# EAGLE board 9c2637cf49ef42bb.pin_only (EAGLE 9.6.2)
REV: D

Size 62.48 x 81.28 mm. Coordinates in mm from the lower left corner, seen from the top.
Outline: 0,2.54 arc90 2.54,0 59.94,0 arc90 62.48,2.54 arc90 59.94,5.08 56.64,5.08 56.64,76.2 59.94,76.2 arc90 62.48,78.74 arc90 59.94,81.28 2.54,81.28 arc90 0,78.74 arc90 2.54,76.2 5.84,76.2 5.84,5.08 2.54,5.08 arc90 0,2.54
Outline: 16.26,24.89 16.26,19.56 37.21,19.56 37.21,6.1 53.21,6.1 53.21,19.56 46.23,19.56 46.23,24.89 16.26,24.89
Copper layers (1*16): Top 0.035mm / dielectric 1.5mm / Bottom 0.035mm
Design rules "adafruit *": minimum track width 8mil, minimum drill 15.5mil, track to track 8mil, track to pad 8mil, pad to pad 8mil, via to via 8mil, smd to smd 8mil, copper to edge 10mil, drill to drill 8mil, minimum pad ring 10mil, minimum via ring 8mil, stop-mask expansion 4mil, vias tented up to drill 20mil, thermal gap 10mil
tRestrict: area 42.7,32.6 to 42.8,32.9; area 43.2,32.6 to 43.3,32.9

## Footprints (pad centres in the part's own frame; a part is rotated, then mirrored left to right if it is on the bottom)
0805-NO = smd 1.24 x 1.5: 1 -0.95,0; 2 0.95,0
TFT_2.83IN_240X320_50PIN = smd 0.275 x 1.2 bottom: 1 12.25,1.04; 2 11.75,1.04; 3 11.25,1.04; 4 10.75,1.04; 5 10.25,1.04; 6 9.75,1.04; 7 9.25,1.04; 8 8.75,1.04; 9 8.25,1.04; 10 7.75,1.04; 11 7.25,1.04; 12 6.75,1.04; 13 6.25,1.04; 14 5.75,1.04; 15 5.25,1.04; 16 4.75,1.04; 17 4.25,1.04; 18 3.75,1.04; 19 3.25,1.04; 20 2.75,1.04; 21 2.25,1.04; 22 1.75,1.04; 23 1.25,1.04; 24 0.75,1.04; 25 0.25,1.04; 26 -0.25,1.04; 27 -0.75,1.04; 28 -1.25,1.04; 29 -1.75,1.04; 30 -2.25,1.04; 31 -2.75,1.04; 32 -3.25,1.04; 33 -3.75,1.04; 34 -4.25,1.04; 35 -4.75,1.04; 36 -5.25,1.04; 37 -5.75,1.04; 38 -6.25,1.04; 39 -6.75,1.04; 40 -7.25,1.04; 41 -7.75,1.04; 42 -8.25,1.04; 43 -8.75,1.04; 44 -9.25,1.04; 45 -9.75,1.04; 46 -10.25,1.04; 47 -10.75,1.04; 48 -11.25,1.04; 49 -11.75,1.04; 50 -12.25,1.04 | smd 2.54 x 3.81 bottom: PAD1 14.35,-1.152; PAD2 -14.35,-1.152
SOT23-WIDE = smd 1 x 1.2: 1 -0.95,-1; 2 0.95,-1; 3 0,1
1X20_ROUND = drill 1 pad 1.676: 1 -24.13,0; 2 -21.59,0; 3 -19.05,0; 4 -16.51,0; 5 -13.97,0; 6 -11.43,0; 7 -8.89,0; 8 -6.35,0; 9 -3.81,0; 10 -1.27,0; 11 1.27,0; 12 3.81,0; 13 6.35,0; 14 8.89,0; 15 11.43,0; 16 13.97,0; 17 16.51,0; 18 19.05,0; 19 21.59,0; 20 24.13,0
0603-NO = smd 1.075 x 1: 1 -0.85,0; 2 0.85,0
SOLDERJUMPER_ARROW_NOPASTE = smd 0.762 x 1.524: 1 -1.016,0; 2 1.016,0
TP06R = smd 0.6 x 0.6: TP 0,0
SOT23-5 = smd 0.55 x 1.2: 1 -0.95,-1.3; 2 0,-1.3; 3 0.95,-1.3; 4 0.95,1.3; 5 -0.95,1.3
TSSOP20 = smd 0.305 x 0.991: 1 -2.925,-2.918; 2 -2.275,-2.918; 3 -1.625,-2.918; 4 -0.975,-2.918; 5 -0.325,-2.918; 6 0.325,-2.918; 7 0.975,-2.918; 8 1.625,-2.918; 9 2.275,-2.918; 10 2.925,-2.918; 11 2.925,2.918; 12 2.275,2.918; 13 1.625,2.918; 14 0.975,2.918; 15 0.325,2.918; 16 -0.325,2.918; 17 -0.975,2.918; 18 -1.625,2.918; 19 -2.275,2.918; 20 -2.925,2.918
MOUNTINGHOLE_3.0_PLATEDTHIN = drill 3 pad 3.6: P$1 0,0
FIDUCIAL_1MM = smd 1 x 1: 1 0,0
EYE_SPI_DISPLAY_BOTCONTACT = smd 0.25 x 1.4: 1 4.25,1.154; 2 3.75,1.154; 3 3.25,1.154; 4 2.75,1.154; 5 2.25,1.154; 6 1.75,1.154; 7 1.25,1.154; 8 0.75,1.154; 9 0.25,1.154; 10 -0.25,1.154; 11 -0.75,1.154; 12 -1.25,1.154; 13 -1.75,1.154; 14 -2.25,1.154; 15 -2.75,1.154; 16 -3.25,1.154; 17 -3.75,1.154; 18 -4.25,1.154 | smd 1.8 x 3.5: SUPPORT1 -5.8,-1.152; SUPPORT2 5.8,-1.152
MICROSD = smd 0.7 x 1.5: 1 1.761,-3.147; 2 0.661,-2.747; 3 -0.439,-3.147; 4 -1.539,-3.547; 5 -2.639,-3.147; 6 -3.739,-3.547; 7 -4.839,-3.147; 8 -5.939,-3.147 | smd 1.8 x 1.4: CD1 -5.239,7.053; CD2 0.38,7.053 | smd 1.4 x 1.9: MT1 -6.839,-6.047; MT2 6.361,-6.947

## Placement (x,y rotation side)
C1  10uF  [0805-NO]  16.26,50.8 0 top
C3  10uF  [0805-NO]  50.04,44.32 0 top
C4  10uF  [0805-NO]  25.91,38.35 270 top
C5  10uF  [0805-NO]  51.44,37.08 270 top
CONN1  2.8" CTP ILI9341  [TFT_2.83IN_240X320_50PIN]  31.24,31.75 0 bottom
IC4  APX803-SAG  [SOT23-WIDE]  36.32,49.78 0 top
JP1  [1X20_ROUND]  31.24,78.74 180 top
JP2  [1X20_ROUND]  31.24,2.54 180 top
PLABEL0  [PLABEL0]  27.43,37.97 0 top
PLABEL1  [PLABEL1]  55.88,17.65 90 top
PLABEL2  [PLABEL2]  26.54,52.7 0 top
PLABEL3  [PLABEL3]  24.64,65.28 0 top
PLABEL4  [PLABEL4]  6.6,77.47 270 top
PLABEL5  [PLABEL5]  8.89,77.47 270 top
PLABEL6  [PLABEL6]  11.43,77.47 270 top
PLABEL7  [PLABEL7]  13.97,77.6 270 top
PLABEL8  [PLABEL8]  16.64,77.72 270 top
PLABEL9  [PLABEL9]  19.18,77.72 270 top
PLABEL10  [PLABEL10]  21.59,77.72 270 top
PLABEL11  [PLABEL11]  24.26,77.72 270 top
PLABEL12  [PLABEL12]  26.8,77.72 270 top
PLABEL13  [PLABEL13]  29.21,77.72 270 top
PLABEL14  [PLABEL14]  31.88,77.72 270 top
PLABEL15  [PLABEL15]  34.29,77.72 270 top
PLABEL16  [PLABEL16]  36.96,77.72 270 top
PLABEL17  [PLABEL17]  39.5,77.72 270 top
PLABEL18  [PLABEL18]  41.91,77.72 270 top
PLABEL19  [PLABEL19]  44.58,77.72 270 top
PLABEL20  [PLABEL20]  47.12,77.72 270 top
PLABEL21  [PLABEL21]  49.53,77.6 270 top
PLABEL22  [PLABEL22]  52.2,77.72 270 top
PLABEL23  [PLABEL23]  54.61,77.72 270 top
PLABEL24  [PLABEL24]  11.18,67.56 0 top
PLABEL25  [PLABEL25]  27.81,68.33 0 top
PLABEL26  [PLABEL26]  39.62,69.85 0 top
PLABEL27  [PLABEL27]  52.58,69.6 0 top
PLABEL28  [PLABEL28]  39.62,68.2 0 top
PLABEL29  [PLABEL29]  11.43,69.6 0 top
PLABEL30  [PLABEL30]  27.3,34.67 0 top
PLABEL31  [PLABEL31]  7.62,3.81 90 top
PLABEL32  [PLABEL32]  10.16,3.81 90 top
PLABEL33  [PLABEL33]  12.7,3.81 90 top
PLABEL34  [PLABEL34]  15.24,3.81 90 top
PLABEL35  [PLABEL35]  17.78,3.81 90 top
PLABEL36  [PLABEL36]  20.32,3.81 90 top
PLABEL37  [PLABEL37]  22.86,3.81 90 top
PLABEL38  [PLABEL38]  25.4,3.81 90 top
PLABEL39  [PLABEL39]  27.94,3.81 90 top
PLABEL40  [PLABEL40]  30.48,3.81 90 top
PLABEL41  [PLABEL41]  33.02,3.81 90 top
PLABEL42  [PLABEL42]  35.56,3.81 90 top
PLABEL43  [PLABEL43]  38.1,3.68 90 top
PLABEL44  [PLABEL44]  40.51,3.68 90 top
PLABEL45  [PLABEL45]  40.89,3.68 0 top
PLABEL46  [PLABEL46]  43.43,0.38 0 top
PLABEL47  [PLABEL47]  46.23,3.68 0 top
PLABEL48  [PLABEL48]  50.8,3.43 90 top
PLABEL49  [PLABEL49]  53.34,3.56 90 top
PLABEL50  [PLABEL50]  56.01,3.56 90 top
PLABEL51  [PLABEL51]  7.75,30.99 0 top
PLABEL52  [PLABEL52]  7.87,34.8 0 top
PLABEL53  [PLABEL53]  7.75,38.73 0 top
PLABEL54  [PLABEL54]  7.75,42.8 0 top
PLABEL55  [PLABEL55]  28.58,14.86 0 top
PLABEL56  [PLABEL56]  13.84,28.96 90 top
PLABEL57  [PLABEL57]  9.65,77.47 0 bottom
PLABEL58  [PLABEL58]  12.19,77.47 0 bottom
PLABEL59  [PLABEL59]  14.73,77.47 0 bottom
PLABEL60  [PLABEL60]  17.27,77.47 0 bottom
PLABEL61  [PLABEL61]  7.11,77.47 0 bottom
PLABEL62  [PLABEL62]  19.81,77.47 0 bottom
PLABEL63  [PLABEL63]  22.35,77.47 0 bottom
PLABEL64  [PLABEL64]  24.89,77.47 0 bottom
PLABEL65  [PLABEL65]  27.3,81.03 0 bottom
PLABEL66  [PLABEL66]  29.97,77.47 0 bottom
PLABEL67  [PLABEL67]  32.64,81.03 0 bottom
PLABEL68  [PLABEL68]  35.05,77.47 0 bottom
PLABEL69  [PLABEL69]  37.59,81.15 0 bottom
PLABEL70  [PLABEL70]  40.13,77.47 0 bottom
PLABEL71  [PLABEL71]  42.8,79.88 180 bottom
PLABEL72  [PLABEL72]  45.21,77.47 0 bottom
PLABEL73  [PLABEL73]  47.62,79.76 180 bottom
PLABEL74  [PLABEL74]  50.29,77.47 0 bottom
PLABEL75  [PLABEL75]  52.83,81.15 0 bottom
PLABEL76  [PLABEL76]  55.37,77.6 0 bottom
PLABEL77  [PLABEL77]  7.11,5.08 0 bottom
PLABEL78  [PLABEL78]  9.65,0.25 0 bottom
PLABEL79  [PLABEL79]  12.19,3.68 0 bottom
PLABEL80  [PLABEL80]  14.73,0.25 0 bottom
PLABEL81  [PLABEL81]  17.27,3.68 0 bottom
PLABEL82  [PLABEL82]  19.81,0.25 0 bottom
PLABEL83  [PLABEL83]  22.35,3.68 0 bottom
PLABEL84  [PLABEL84]  24.89,0.25 0 bottom
PLABEL85  [PLABEL85]  27.43,3.68 0 bottom
PLABEL86  [PLABEL86]  29.97,0.25 0 bottom
PLABEL87  [PLABEL87]  32.51,3.68 0 bottom
PLABEL88  [PLABEL88]  35.05,0.25 0 bottom
PLABEL89  [PLABEL89]  37.59,3.56 0 bottom
PLABEL90  [PLABEL90]  40.26,0.25 0 bottom
PLABEL91  [PLABEL91]  42.67,3.68 0 bottom
PLABEL92  [PLABEL92]  45.09,0.25 0 bottom
PLABEL93  [PLABEL93]  47.75,3.68 0 bottom
PLABEL94  [PLABEL94]  50.29,0.25 0 bottom
PLABEL95  [PLABEL95]  52.83,3.56 0 bottom
PLABEL96  [PLABEL96]  55.37,0.25 0 bottom
Q2  BSS138  [SOT23-WIDE]  22.35,10.92 180 top
Q3  BSS138  [SOT23-WIDE]  26.29,10.92 180 top
Q4  BSS138  [SOT23-WIDE]  14.48,37.47 0 top
R1  10  [0603-NO]  17.53,38.35 270 top
R2  10  [0603-NO]  19.56,38.35 270 top
R3  10  [0603-NO]  21.59,38.35 270 top
R4  10  [0603-NO]  23.62,38.35 270 top
R5  2.2K  [0603-NO]  14.22,40.89 180 top
R6  10K  [0603-NO]  38.86,49.78 90 top
R7  1K  [0603-NO]  37.85,68.07 0 top
R8  10K  [0603-NO]  8.76,13.21 90 top
R9  10K  [0603-NO]  11.18,12.57 90 top
R10  10K  [0603-NO]  16.38,12.57 270 top
R11  10K  [0603-NO]  13.72,12.57 270 top
R12  10K  [0603-NO]  37.47,62.87 270 top
R13  10K  [0603-NO]  22.48,8.26 0 top
R14  10K  [0603-NO]  26.29,8.26 180 top
R15  10K  [0603-NO]  26.29,13.72 180 top
R16  10K  [0603-NO]  22.35,13.72 0 top
SJ1  [SOLDERJUMPER_ARROW_NOPASTE]  8.89,29.72 180 top
SJ2  [SOLDERJUMPER_ARROW_NOPASTE]  8.89,33.53 180 top
SJ3  [SOLDERJUMPER_ARROW_NOPASTE]  8.89,37.47 0 top
SJ4  [SOLDERJUMPER_ARROW_NOPASTE]  8.89,41.53 0 top
TFT1  2.8in CTP TFT  [TP06R]  31.24,30.48 0 top
U1  AP2112K-3.3  [SOT23-5]  50.8,40.89 0 top
U2  74LVC245  [TSSOP20]  43.69,58.8 180 top
U3  74LVC245  [TSSOP20]  31.5,59.18 180 top
U$7  MOUNTINGHOLE3.0THIN  [MOUNTINGHOLE_3.0_PLATEDTHIN]  2.67,2.54 0 top
U$9  FIDUCIAL  [FIDUCIAL_1MM]  49.78,22.86 0 top
U$11  FIDUCIAL  [FIDUCIAL_1MM]  8.89,69.09 0 top
U$15  MOUNTINGHOLE3.0THIN  [MOUNTINGHOLE_3.0_PLATEDTHIN]  59.82,2.54 0 top
U$16  MOUNTINGHOLE3.0THIN  [MOUNTINGHOLE_3.0_PLATEDTHIN]  2.67,78.74 0 top
U$17  MOUNTINGHOLE3.0THIN  [MOUNTINGHOLE_3.0_PLATEDTHIN]  59.82,78.74 0 top
U$19  [ADAFRUIT_TEXT_30MM]  14.1,40.26 0 top
U$23  FIDUCIAL  [FIDUCIAL_1MM]  15.24,33.78 0 top
U$28  [PCBFEAT-REV-040]  45.85,35.69 0 top
U$29  [EYESPI_MINI_LOGO]  55.5,46.1 90 top
X1  EYE_SPI_DISPLAY_FLIP  [EYE_SPI_DISPLAY_BOTCONTACT]  52.2,59.05 90 top
X2  MicroSD  [MICROSD]  15.37,59.05 270 top

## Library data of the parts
C1 C3-C5 JP1 JP2 R1-R13 R15 R16 U2 U3 U$19 = microbuilder
CONN1 = adafruit_display
IC4 Q2-Q4 R14 = microbuilder; ROT: 270
PLABEL0 PLABEL1-PLABEL96 = pinguin
SJ1-SJ4 = microbuilder; BOM: EXCLUDE
TFT1 = testpad
U1 = adafruit_power; JLC_ROTATION: 0
U$7 U$15-U$17 = adafruit_electromech; BOM: EXCLUDE
U$9 U$11 U$23 = adafruit
U$28 = microbuilder; REV: D
U$29 = silks
X1 = adafruit_display; LCSC: C2856802
X2 = adafruit_electromech; JLC_ROTATION: 90; LCSC: C125617

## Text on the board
Pinguin_tBackup: D7 | D6 | D5 | D4 | D3 | D2 | D1 | D0 | GND | SDA | SCL | IRQ | Backlite | RST | RD | WR | C/D | CS | 3-5V | GND | LCD Data I/O | LCD control | PWR | Capacitive / Touchscreen | Inputs | Bi-directional | 8-bit 8080-type parallel | Logic:3V-5V | IM3 | IM2 | 2.8" TFT ILI9341 | I2C CapTouch | IM1 | IM0 | Close IM1/IM2/IM3 / for SPI | SPI Interface | Vin:3.3V-5V | MISO | Card Detect | Card CS | IM0 | IM1 | IM2 | IM3 | SCL | SDA | IRQ | GND | Lite | RST | DC | CS | 3Vo | Vin | GND | MOSI | CLK
Pinguin_bBackup: GND | SCL | Lite | RD | C/D | Vin | D7 | D6 | D5 | D4 | D3 | D2 | D1 | D0 | SDA | IRQ | RST | WR | CS | GND | CD | IM0 | IM2 | SCL | IRQ | Lite | D/C | MOSI | CLK | Vin | CCS | IM1 | IM3 | SDA | GND | RST | CS | MISO | 3Vo | GND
